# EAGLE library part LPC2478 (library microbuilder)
LPC2470/2478 - ARM7TDMI-S 72MHz MCU Single-chip 16-bit/32-bit micro; 512 kB flash, Ethernet, CAN, LCD, USB 2.0 device/host/OTG, external memory interface Digikey: 568-4363-ND
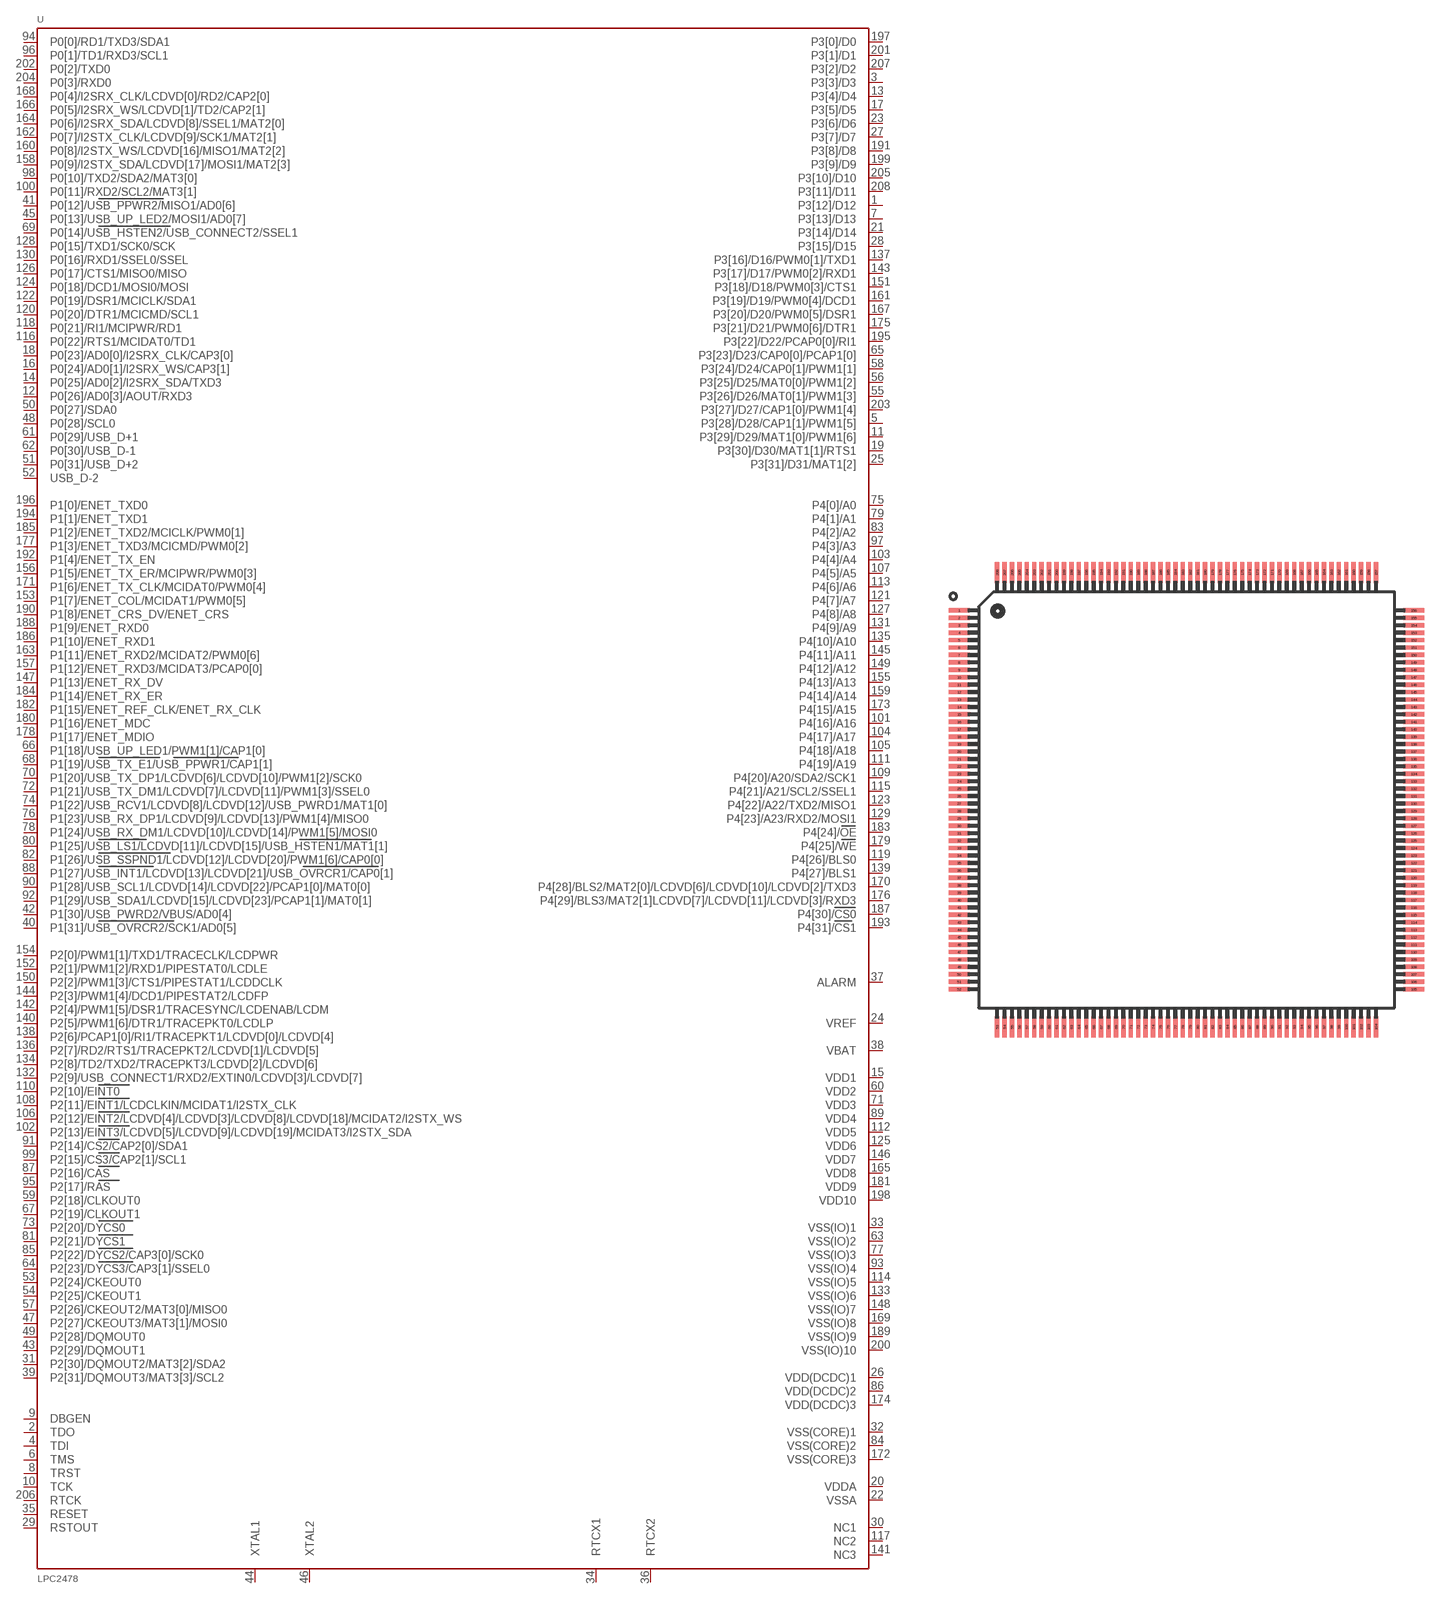
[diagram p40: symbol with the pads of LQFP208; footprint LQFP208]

Designator prefix U

## LPC2478  [LQFP208]
1  P3[12]/D12
2  TDO
3  P3[3]/D3
4  TDI
5  P3[28]/D28/CAP1[1]/PWM1[5]
6  TMS
7  P3[13]/D13
8  TRST
9  DBGEN
10  TCK
11  P3[29]/D29/MAT1[0]/PWM1[6]
12  P0[26]/AD0[3]/AOUT/RXD3
13  P3[4]/D4
14  P0[25]/AD0[2]/I2SRX_SDA/TXD3
15  VDD1
16  P0[24]/AD0[1]/I2SRX_WS/CAP3[1]
17  P3[5]/D5
18  P0[23]/AD0[0]/I2SRX_CLK/CAP3[0]
19  P3[30]/D30/MAT1[1]/RTS1
20  VDDA
21  P3[14]/D14
22  VSSA
23  P3[6]/D6
24  VREF
25  P3[31]/D31/MAT1[2]
26  VDD(DCDC)1
27  P3[7]/D7
28  P3[15]/D15
29  RSTOUT
30  NC1
31  P2[30]/DQMOUT2/MAT3[2]/SDA2
32  VSS(CORE)1
33  VSS(IO)1
34  RTCX1
35  RESET
36  RTCX2
37  ALARM
38  VBAT
39  P2[31]/DQMOUT3/MAT3[3]/SCL2
40  P1[31]/USB_OVRCR2/SCK1/AD0[5]
41  P0[12]/USB_PPWR2/MISO1/AD0[6]
42  P1[30]/USB_PWRD2/VBUS/AD0[4]
43  P2[29]/DQMOUT1
44  XTAL1
45  P0[13]/USB_UP_LED2/MOSI1/AD0[7]
46  XTAL2
47  P2[27]/CKEOUT3/MAT3[1]/MOSI0
48  P0[28]/SCL0
49  P2[28]/DQMOUT0
50  P0[27]/SDA0
51  P0[31]/USB_D+2
52  USB_D-2
53  P2[24]/CKEOUT0
54  P2[25]/CKEOUT1
55  P3[26]/D26/MAT0[1]/PWM1[3]
56  P3[25]/D25/MAT0[0]/PWM1[2]
57  P2[26]/CKEOUT2/MAT3[0]/MISO0
58  P3[24]/D24/CAP0[1]/PWM1[1]
59  P2[18]/CLKOUT0
60  VDD2
61  P0[29]/USB_D+1
62  P0[30]/USB_D-1
63  VSS(IO)2
64  P2[23]/DYCS3/CAP3[1]/SSEL0
65  P3[23]/D23/CAP0[0]/PCAP1[0]
66  P1[18]/USB_UP_LED1/PWM1[1]/CAP1[0]
67  P2[19]/CLKOUT1
68  P1[19]/USB_TX_E1/USB_PPWR1/CAP1[1]
69  P0[14]/USB_HSTEN2/USB_CONNECT2/SSEL1
70  P1[20]/USB_TX_DP1/LCDVD[6]/LCDVD[10]/PWM1[2]/SCK0
71  VDD3
72  P1[21]/USB_TX_DM1/LCDVD[7]/LCDVD[11]/PWM1[3]/SSEL0
73  P2[20]/DYCS0
74  P1[22]/USB_RCV1/LCDVD[8]/LCDVD[12]/USB_PWRD1/MAT1[0]
75  P4[0]/A0
76  P1[23]/USB_RX_DP1/LCDVD[9]/LCDVD[13]/PWM1[4]/MISO0
77  VSS(IO)3
78  P1[24]/USB_RX_DM1/LCDVD[10]/LCDVD[14]/PWM1[5]/MOSI0
79  P4[1]/A1
80  P1[25]/USB_LS1/LCDVD[11]/LCDVD[15]/USB_HSTEN1/MAT1[1]
81  P2[21]/DYCS1
82  P1[26]/USB_SSPND1/LCDVD[12]/LCDVD[20]/PWM1[6]/CAP0[0]
83  P4[2]/A2
84  VSS(CORE)2
85  P2[22]/DYCS2/CAP3[0]/SCK0
86  VDD(DCDC)2
87  P2[16]/CAS
88  P1[27]/USB_INT1/LCDVD[13]/LCDVD[21]/USB_OVRCR1/CAP0[1]
89  VDD4
90  P1[28]/USB_SCL1/LCDVD[14]/LCDVD[22]/PCAP1[0]/MAT0[0]
91  P2[14]/CS2/CAP2[0]/SDA1
92  P1[29]/USB_SDA1/LCDVD[15]/LCDVD[23]/PCAP1[1]/MAT0[1]
93  VSS(IO)4
94  P0[0]/RD1/TXD3/SDA1
95  P2[17]/RAS
96  P0[1]/TD1/RXD3/SCL1
97  P4[3]/A3
98  P0[10]/TXD2/SDA2/MAT3[0]
99  P2[15]/CS3/CAP2[1]/SCL1
100  P0[11]/RXD2/SCL2/MAT3[1]
101  P4[16]/A16
102  P2[13]/EINT3/LCDVD[5]/LCDVD[9]/LCDVD[19]/MCIDAT3/I2STX_SDA
103  P4[4]/A4
104  P4[17]/A17
105  P4[18]/A18
106  P2[12]/EINT2/LCDVD[4]/LCDVD[3]/LCDVD[8]/LCDVD[18]/MCIDAT2/I2STX_WS
107  P4[5]/A5
108  P2[11]/EINT1/LCDCLKIN/MCIDAT1/I2STX_CLK
109  P4[20]/A20/SDA2/SCK1
110  P2[10]/EINT0
111  P4[19]/A19
112  VDD5
113  P4[6]/A6
114  VSS(IO)5
115  P4[21]/A21/SCL2/SSEL1
116  P0[22]/RTS1/MCIDAT0/TD1
117  NC2
118  P0[21]/RI1/MCIPWR/RD1
119  P4[26]/BLS0
120  P0[20]/DTR1/MCICMD/SCL1
121  P4[7]/A7
122  P0[19]/DSR1/MCICLK/SDA1
123  P4[22]/A22/TXD2/MISO1
124  P0[18]/DCD1/MOSI0/MOSI
125  VDD6
126  P0[17]/CTS1/MISO0/MISO
127  P4[8]/A8
128  P0[15]/TXD1/SCK0/SCK
129  P4[23]/A23/RXD2/MOSI1
130  P0[16]/RXD1/SSEL0/SSEL
131  P4[9]/A9
132  P2[9]/USB_CONNECT1/RXD2/EXTIN0/LCDVD[3]/LCDVD[7]
133  VSS(IO)6
134  P2[8]/TD2/TXD2/TRACEPKT3/LCDVD[2]/LCDVD[6]
135  P4[10]/A10
136  P2[7]/RD2/RTS1/TRACEPKT2/LCDVD[1]/LCDVD[5]
137  P3[16]/D16/PWM0[1]/TXD1
138  P2[6]/PCAP1[0]/RI1/TRACEPKT1/LCDVD[0]/LCDVD[4]
139  P4[27]/BLS1
140  P2[5]/PWM1[6]/DTR1/TRACEPKT0/LCDLP
141  NC3
142  P2[4]/PWM1[5]/DSR1/TRACESYNC/LCDENAB/LCDM
143  P3[17]/D17/PWM0[2]/RXD1
144  P2[3]/PWM1[4]/DCD1/PIPESTAT2/LCDFP
145  P4[11]/A11
146  VDD7
147  P1[13]/ENET_RX_DV
148  VSS(IO)7
149  P4[12]/A12
150  P2[2]/PWM1[3]/CTS1/PIPESTAT1/LCDDCLK
151  P3[18]/D18/PWM0[3]/CTS1
152  P2[1]/PWM1[2]/RXD1/PIPESTAT0/LCDLE
153  P1[7]/ENET_COL/MCIDAT1/PWM0[5]
154  P2[0]/PWM1[1]/TXD1/TRACECLK/LCDPWR
155  P4[13]/A13
156  P1[5]/ENET_TX_ER/MCIPWR/PWM0[3]
157  P1[12]/ENET_RXD3/MCIDAT3/PCAP0[0]
158  P0[9]/I2STX_SDA/LCDVD[17]/MOSI1/MAT2[3]
159  P4[14]/A14
160  P0[8]/I2STX_WS/LCDVD[16]/MISO1/MAT2[2]
161  P3[19]/D19/PWM0[4]/DCD1
162  P0[7]/I2STX_CLK/LCDVD[9]/SCK1/MAT2[1]
163  P1[11]/ENET_RXD2/MCIDAT2/PWM0[6]
164  P0[6]/I2SRX_SDA/LCDVD[8]/SSEL1/MAT2[0]
165  VDD8
166  P0[5]/I2SRX_WS/LCDVD[1]/TD2/CAP2[1]
167  P3[20]/D20/PWM0[5]/DSR1
168  P0[4]/I2SRX_CLK/LCDVD[0]/RD2/CAP2[0]
169  VSS(IO)8
170  P4[28]/BLS2/MAT2[0]/LCDVD[6]/LCDVD[10]/LCDVD[2]/TXD3
171  P1[6]/ENET_TX_CLK/MCIDAT0/PWM0[4]
172  VSS(CORE)3
173  P4[15]/A15
174  VDD(DCDC)3
175  P3[21]/D21/PWM0[6]/DTR1
176  P4[29]/BLS3/MAT2[1]LCDVD[7]/LCDVD[11]/LCDVD[3]/RXD3
177  P1[3]/ENET_TXD3/MCICMD/PWM0[2]
178  P1[17]/ENET_MDIO
179  P4[25]/WE
180  P1[16]/ENET_MDC
181  VDD9
182  P1[15]/ENET_REF_CLK/ENET_RX_CLK
183  P4[24]/OE
184  P1[14]/ENET_RX_ER
185  P1[2]/ENET_TXD2/MCICLK/PWM0[1]
186  P1[10]/ENET_RXD1
187  P4[30]/CS0
188  P1[9]/ENET_RXD0
189  VSS(IO)9
190  P1[8]/ENET_CRS_DV/ENET_CRS
191  P3[8]/D8
192  P1[4]/ENET_TX_EN
193  P4[31]/CS1
194  P1[1]/ENET_TXD1
195  P3[22]/D22/PCAP0[0]/RI1
196  P1[0]/ENET_TXD0
197  P3[0]/D0
198  VDD10
199  P3[9]/D9
200  VSS(IO)10
201  P3[1]/D1
202  P0[2]/TXD0
203  P3[27]/D27/CAP1[0]/PWM1[4]
204  P0[3]/RXD0
205  P3[10]/D10
206  RTCK
207  P3[2]/D2
208  P3[11]/D11

## Footprint LQFP208 (pad centres in mm)
smd 1.4 x 0.29: 1 -15.3,12.75; 2 -15.3,12.25; 3 -15.3,11.75; 4 -15.3,11.25; 5 -15.3,10.75; 6 -15.3,10.25; 7 -15.3,9.75; 8 -15.3,9.25; 9 -15.3,8.75; 10 -15.3,8.25; 11 -15.3,7.75; 12 -15.3,7.25; 13 -15.3,6.75; 14 -15.3,6.25; 15 -15.3,5.75; 16 -15.3,5.25; 17 -15.3,4.75; 18 -15.3,4.25; 19 -15.3,3.75; 20 -15.3,3.25; 21 -15.3,2.75; 22 -15.3,2.25; 23 -15.3,1.75; 24 -15.3,1.25; 25 -15.3,0.75; 26 -15.3,0.25; 27 -15.3,-0.25; 28 -15.3,-0.75; 29 -15.3,-1.25; 30 -15.3,-1.75; 31 -15.3,-2.25; 32 -15.3,-2.75; 33 -15.3,-3.25; 34 -15.3,-3.75; 35 -15.3,-4.25; 36 -15.3,-4.75; 37 -15.3,-5.25; 38 -15.3,-5.75; 39 -15.3,-6.25; 40 -15.3,-6.75; 41 -15.3,-7.25; 42 -15.3,-7.75; 43 -15.3,-8.25; 44 -15.3,-8.75; 45 -15.3,-9.25; 46 -15.3,-9.75; 47 -15.3,-10.25; 48 -15.3,-10.75; 49 -15.3,-11.25; 50 -15.3,-11.75; 51 -15.3,-12.25; 52 -15.3,-12.75; 105 15.3,-12.75; 106 15.3,-12.25; 107 15.3,-11.75; 108 15.3,-11.25; 109 15.3,-10.75; 110 15.3,-10.25; 111 15.3,-9.75; 112 15.3,-9.25; 113 15.3,-8.75; 114 15.3,-8.25; 115 15.3,-7.75; 116 15.3,-7.25; 117 15.3,-6.75; 118 15.3,-6.25; 119 15.3,-5.75; 120 15.3,-5.25; 121 15.3,-4.75; 122 15.3,-4.25; 123 15.3,-3.75; 124 15.3,-3.25; 125 15.3,-2.75; 126 15.3,-2.25; 127 15.3,-1.75; 128 15.3,-1.25; 129 15.3,-0.75; 130 15.3,-0.25; 131 15.3,0.25; 132 15.3,0.75; 133 15.3,1.25; 134 15.3,1.75; 135 15.3,2.25; 136 15.3,2.75; 137 15.3,3.25; 138 15.3,3.75; 139 15.3,4.25; 140 15.3,4.75; 141 15.3,5.25; 142 15.3,5.75; 143 15.3,6.25; 144 15.3,6.75; 145 15.3,7.25; 146 15.3,7.75; 147 15.3,8.25; 148 15.3,8.75; 149 15.3,9.25; 150 15.3,9.75; 151 15.3,10.25; 152 15.3,10.75; 153 15.3,11.25; 154 15.3,11.75; 155 15.3,12.25; 156 15.3,12.75
smd 0.29 x 1.4: 53 -12.75,-15.3; 54 -12.25,-15.3; 55 -11.75,-15.3; 56 -11.25,-15.3; 57 -10.75,-15.3; 58 -10.25,-15.3; 59 -9.75,-15.3; 60 -9.25,-15.3; 61 -8.75,-15.3; 62 -8.25,-15.3; 63 -7.75,-15.3; 64 -7.25,-15.3; 65 -6.75,-15.3; 66 -6.25,-15.3; 67 -5.75,-15.3; 68 -5.25,-15.3; 69 -4.75,-15.3; 70 -4.25,-15.3; 71 -3.75,-15.3; 72 -3.25,-15.3; 73 -2.75,-15.3; 74 -2.25,-15.3; 75 -1.75,-15.3; 76 -1.25,-15.3; 77 -0.75,-15.3; 78 -0.25,-15.3; 79 0.25,-15.3; 80 0.75,-15.3; 81 1.25,-15.3; 82 1.75,-15.3; 83 2.25,-15.3; 84 2.75,-15.3; 85 3.25,-15.3; 86 3.75,-15.3; 87 4.25,-15.3; 88 4.75,-15.3; 89 5.25,-15.3; 90 5.75,-15.3; 91 6.25,-15.3; 92 6.75,-15.3; 93 7.25,-15.3; 94 7.75,-15.3; 95 8.25,-15.3; 96 8.75,-15.3; 97 9.25,-15.3; 98 9.75,-15.3; 99 10.25,-15.3; 100 10.75,-15.3; 101 11.25,-15.3; 102 11.75,-15.3; 103 12.25,-15.3; 104 12.75,-15.3; 157 12.75,15.3; 158 12.25,15.3; 159 11.75,15.3; 160 11.25,15.3; 161 10.75,15.3; 162 10.25,15.3; 163 9.75,15.3; 164 9.25,15.3; 165 8.75,15.3; 166 8.25,15.3; 167 7.75,15.3; 168 7.25,15.3; 169 6.75,15.3; 170 6.25,15.3; 171 5.75,15.3; 172 5.25,15.3; 173 4.75,15.3; 174 4.25,15.3; 175 3.75,15.3; 176 3.25,15.3; 177 2.75,15.3; 178 2.25,15.3; 179 1.75,15.3; 180 1.25,15.3; 181 0.75,15.3; 182 0.25,15.3; 183 -0.25,15.3; 184 -0.75,15.3; 185 -1.25,15.3; 186 -1.75,15.3; 187 -2.25,15.3; 188 -2.75,15.3; 189 -3.25,15.3; 190 -3.75,15.3; 191 -4.25,15.3; 192 -4.75,15.3; 193 -5.25,15.3; 194 -5.75,15.3; 195 -6.25,15.3; 196 -6.75,15.3; 197 -7.25,15.3; 198 -7.75,15.3; 199 -8.25,15.3; 200 -8.75,15.3; 201 -9.25,15.3; 202 -9.75,15.3; 203 -10.25,15.3; 204 -10.75,15.3; 205 -11.25,15.3; 206 -11.75,15.3; 207 -12.25,15.3; 208 -12.75,15.3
